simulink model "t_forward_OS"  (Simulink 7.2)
settings: Solver=ode3  SolverMode=SingleTasking  StartTime=0.0  StopTime=0.01  FixedStep=10e-6  MaxStep=5e-6  RelTol=1e-6  AbsTol=1e-6

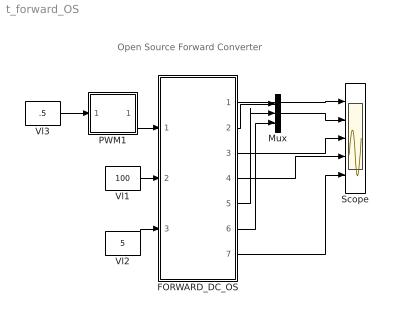
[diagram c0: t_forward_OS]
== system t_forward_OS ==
  note: Open Source Forward Converter
  FORWARD_DC_OS : Subsystem  mask{L1=2e-3, L2=4*2e-3, L3=2e-3, KP1=1, KP2=1, KP3=1, L=1e-3, C=5e-4, UC0=100, R=5}
      mask prompts: L1 "Inductance L1"; L2 "Inductance L2"; L3 "Inductance L3"; KP1 "Coupling Coeff KP12"; KP2 "Coupling Coeff KP23"; KP3 "Coupling Coeff KP31"; L "Inductance"; C "Cap"; UC0 "initial Cap Voltage"; R "Load Resistance"
      mask help: Open Source forward Converter Input Vector u: u[0]= T1.gate u[1]= E.v u[2]= IDC.i Output Vector y: y[0]= T1.I y[1]= D1.I y[2]= L1.I y[3]= Mut_L1.V y[4]= Mut_L2.V y[5]= Mut_L3.V y[6]= D2.I y[7]= D3.I y[8]= C1.V Parameter Vector p: p[0]= Mut_L1.L1 p[1]= Mut_L2.L2 p[2]= Mut_L3.L3 p[3]= Mut_Coupling Coeff.k12 p[4]= Mut_Coupling Coeff.k23 p[5]= Mut_Coupling Coeff.k31 p[6]= L1.L p[7]= C1.C p[8]= C1.vC0 p[9]= R1.r You can pause the simulation during running, change the Parameters you want and continue the Simulation
  Mux : Mux  Inputs=3
  PWM1 : Subsystem  mask(PWMtr){FS=2.5e3}
      mask prompts: FS "Frequency"
  Scope : Scope  NumInputPorts=5
  Vl1 : Constant  Value=100
  Vl2 : Constant  Value=5
  Vl3 : Constant  Value=.5
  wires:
  Vl3/1 -> PWM1/1(In1)
  PWM1/1(Out1) -> FORWARD_DC_OS/1(sw)
  Vl1/1 -> FORWARD_DC_OS/2(E)
  FORWARD_DC_OS/1(iT1) -> Scope/1
  FORWARD_DC_OS/3(iL1) -> Scope/3
  FORWARD_DC_OS/4(vL1,vL2,vL3) -> Scope/4
  Vl2/1 -> FORWARD_DC_OS/3(IDC)
  FORWARD_DC_OS/2(iD1) -> Mux/1
  FORWARD_DC_OS/5(iD2) -> Mux/2
  FORWARD_DC_OS/6(iD3) -> Mux/3
  Mux/1 -> Scope/2
  FORWARD_DC_OS/7(vC) -> Scope/5

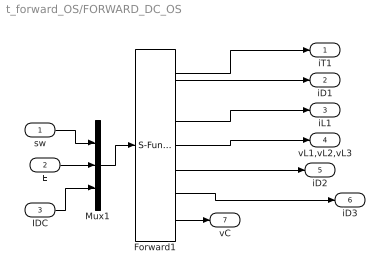
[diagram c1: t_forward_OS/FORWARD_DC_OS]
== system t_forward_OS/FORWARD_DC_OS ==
  sw : Inport  OutDataType=sfix(16)  OutScaling=2^0
  E : Inport  Port=2  OutDataType=sfix(16)  OutScaling=2^0
  IDC : Inport  Port=3  OutDataType=sfix(16)  OutScaling=2^0
  Forward1 : S-Function  FunctionName=s_forward_OS  Parameters="[L1  L2  L3   KP1  KP2  KP3  L C  UC0  R]"  EnableBusSupport=off
  Mux1 : Mux  Inputs=3
  iT1 : Outport  OutDataType=sfix(16)  OutScaling=2^0
  iD1 : Outport  Port=2  OutDataType=sfix(16)  OutScaling=2^0
  iL1 : Outport  Port=3  OutDataType=sfix(16)  OutScaling=2^0
  vL1,vL2,vL3 : Outport  Port=4  OutDataType=sfix(16)  OutScaling=2^0
  iD2 : Outport  Port=5  OutDataType=sfix(16)  OutScaling=2^0
  iD3 : Outport  Port=6  OutDataType=sfix(16)  OutScaling=2^0
  vC : Outport  Port=7  OutDataType=sfix(16)  OutScaling=2^0
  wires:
  sw/1 -> Mux1/1
  Mux1/1 -> Forward1/1
  E/1 -> Mux1/2
  IDC/1 -> Mux1/3
  Forward1/6 -> iD3/1
  Forward1/1 -> iT1/1
  Forward1/2 -> iD1/1
  Forward1/3 -> iL1/1
  Forward1/4 -> vL1,vL2,vL3/1
  Forward1/5 -> iD2/1
  Forward1/7 -> vC/1

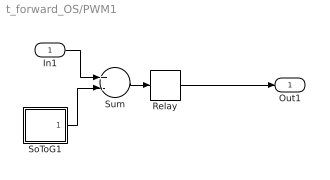
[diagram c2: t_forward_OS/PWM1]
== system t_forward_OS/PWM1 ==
  In1 : Inport
  Relay : Relay
  SoToG1 : Subsystem  mask(SoToG){T=1e-3}
      mask prompts: T "Period Time"
  Sum : Sum  Inputs=+-
  Out1 : Outport  InitialOutput=0
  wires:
  Relay/1 -> Out1/1
  SoToG1/1(O) -> Sum/2
  In1/1 -> Sum/1
  Sum/1 -> Relay/1

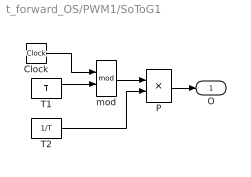
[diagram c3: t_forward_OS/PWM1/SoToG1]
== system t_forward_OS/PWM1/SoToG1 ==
  Clock : Clock
  P : Product
  T1 : Constant  Value=T
  T2 : Constant  Value=1/T
  mod : Math  Operator=mod
  O : Outport
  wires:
  Clock/1 -> mod/1
  T1/1 -> mod/2
  T2/1 -> P/2
  mod/1 -> P/1
  P/1 -> O/1
